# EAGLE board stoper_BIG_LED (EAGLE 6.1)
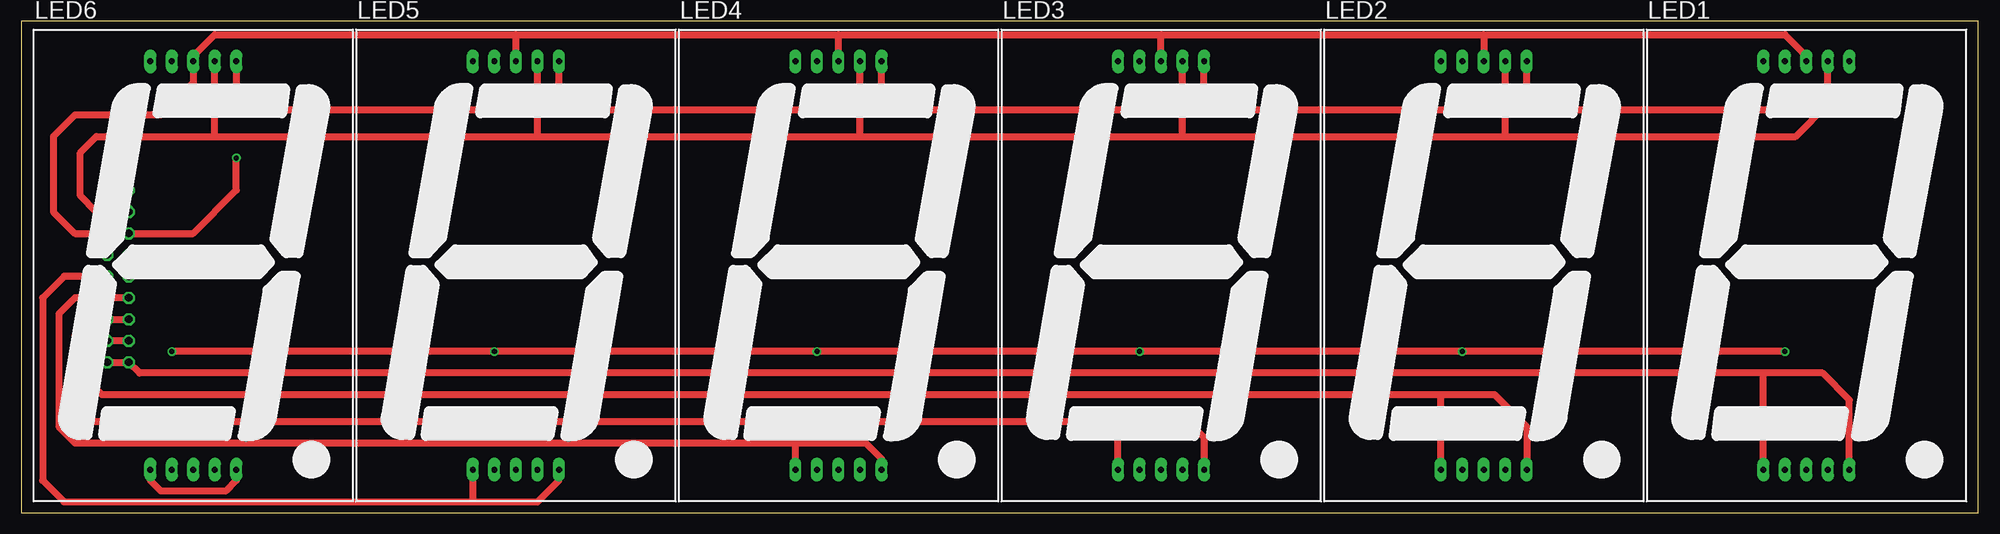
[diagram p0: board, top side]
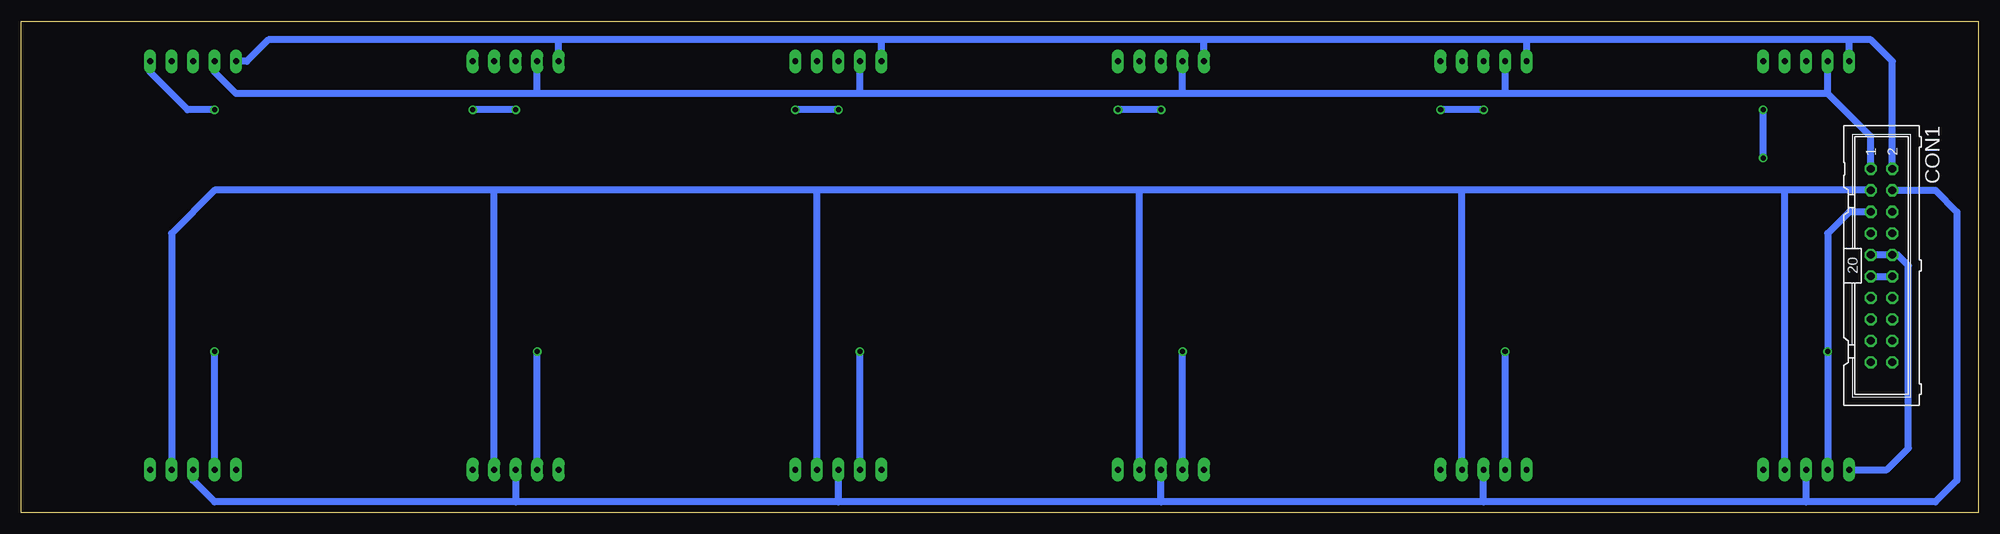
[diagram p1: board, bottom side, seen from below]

Size 231.12 x 58.09 mm. Coordinates in mm from the lower left corner, seen from the top.
Outline: 0,0 231.12,0 231.12,58.09 0,58.09 0,0
Copper layers (1*16): Top 0.035mm / dielectric 1.5mm / Bottom 0.035mm
Design rules: minimum track width 10mil, minimum drill 24mil, track to track 8mil, track to pad 8mil, pad to pad 8mil, via to via 8mil, smd to smd 8mil, copper to edge 40mil, drill to drill 8mil, minimum pad ring 10mil, minimum via ring 8mil, stop-mask expansion 4mil, vias tented up to drill 0mil, thermal gap 10mil

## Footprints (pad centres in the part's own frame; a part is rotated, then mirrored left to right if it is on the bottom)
ML20 = drill 0.914 octagon: 1 -11.43,-1.27; 2 -11.43,1.27; 3 -8.89,-1.27; 4 -8.89,1.27; 5 -6.35,-1.27; 6 -6.35,1.27; 7 -3.81,-1.27; 8 -3.81,1.27; 9 -1.27,-1.27; 10 -1.27,1.27; 11 1.27,-1.27; 12 1.27,1.27; 13 3.81,-1.27; 14 3.81,1.27; 15 6.35,-1.27; 16 6.35,1.27; 17 8.89,-1.27; 18 8.89,1.27; 19 11.43,-1.27; 20 11.43,1.27
SA18-11 = drill 0.7 pad 1.422 long: 1 -5.08,-24.13; 2 -2.54,-24.13; 3 0,-24.13; 4 2.54,-24.13; 5 5.08,-24.13; 6 -5.08,24.13; 7 -2.54,24.13; 8 0,24.13; 9 2.54,24.13; 10 5.08,24.13

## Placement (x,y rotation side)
CON1  [ML20]  11.43,29.21 270 bottom
LED1  7-SEG_SA18-11  [SA18-11]  210.82,29.21 0 top
LED2  7-SEG_SA18-11  [SA18-11]  172.72,29.21 0 top
LED3  7-SEG_SA18-11  [SA18-11]  134.62,29.21 0 top
LED4  7-SEG_SA18-11  [SA18-11]  96.52,29.21 0 top
LED5  7-SEG_SA18-11  [SA18-11]  58.42,29.21 0 top
LED6  7-SEG_SA18-11  [SA18-11]  20.32,29.21 0 top

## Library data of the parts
CON1 = con-harting-ml; OC_FARNELL: unknown; OC_NEWARK: unknown
LED1-LED6 = display-kingbright; OC_FARNELL: unknown; OC_NEWARK: unknown

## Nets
2W1: CON1.19 CON1.20 LED1.1 LED1.5
2W2: CON1.17 CON1.18 LED2.1 LED2.5
2W3: CON1.15 CON1.16 LED3.1 LED3.5
2W4: CON1.13 CON1.14 LED4.1 LED4.5
2W5: CON1.11 CON1.12 LED5.1 LED5.5
2W6: CON1.9 CON1.10 LED6.1 LED6.5
A: CON1.1 LED1.7 LED2.7 LED3.7 LED4.7 LED5.7 LED6.7
B: CON1.2 LED1.6 LED2.6 LED3.6 LED4.6 LED5.6 LED6.6
C: CON1.3 LED1.4 LED2.4 LED3.4 LED4.4 LED5.4 LED6.4
D: CON1.4 LED1.3 LED2.3 LED3.3 LED4.3 LED5.3 LED6.3
DP: CON1.8 LED1.8 LED2.8 LED3.8 LED4.8 LED5.8 LED6.8
E: CON1.5 LED1.2 LED2.2 LED3.2 LED4.2 LED5.2 LED6.2
F: CON1.6 LED1.9 LED2.9 LED3.9 LED4.9 LED5.9 LED6.9
G: CON1.7 LED1.10 LED2.10 LED3.10 LED4.10 LED5.10 LED6.10

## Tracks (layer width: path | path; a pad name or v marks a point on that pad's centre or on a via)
2W1
  Top 0.813: LED1.5 215.9,13.33 212.73,16.51 205.74,16.51 | LED1.1 205.74,16.51 | 205.74,16.51 13.97,16.51 CON1.19 CON1.20
2W2
  Top 0.813: CON1.17 CON1.18 9.53,20.32 8.26,19.05 8.26,15.24 9.53,13.97 167.64,13.97 | 167.64,13.97 173.99,13.97 177.8,10.16 LED2.5 | LED2.1 167.64,13.97
2W3
  Top 0.813: CON1.15 CON1.16 8.26,22.86 6.35,20.95 6.35,12.7 8.26,10.79 129.54,10.79 | 129.54,10.79 137.8,10.79 139.7,8.89 LED3.5 | LED3.1 129.54,10.79
2W4
  Top 0.813: CON1.13 CON1.14 6.35,25.4 4.45,23.5 4.45,10.16 6.35,8.26 91.44,8.26 | 91.44,8.26 99.69,8.26 101.6,6.35 LED4.5 | LED4.1 91.44,8.26
2W5
  Top 0.813: CON1.12 5.08,27.94 2.54,25.4 2.54,3.81 5.08,1.27 53.34,1.27 | 53.34,1.27 60.96,1.27 63.5,3.81 LED5.5 | LED5.1 53.34,1.27
  Bottom 0.813: CON1.11 CON1.12
2W6
  Top 0.813: LED6.5 25.4,3.81 24.13,2.54 16.51,2.54 15.24,3.81 LED6.1
  Bottom 0.813: LED6.1 10.79,5.08 8.26,7.62 8.26,29.21 9.53,30.48 CON1.10 CON1.9
A
  Bottom 0.813: CON1.1 12.7,44.45 17.78,49.53 | 17.78,49.53 LED6.7 | 17.78,49.53 55.88,49.53 | 55.88,49.53 93.98,49.53 | 93.98,49.53 132.08,49.53 | 132.08,49.53 170.18,49.53 | 170.18,49.53 205.74,49.53 208.28,52.07 LED1.7 | 170.18,49.53 LED2.7 | 132.08,49.53 LED3.7 | 93.98,49.53 LED4.7 | 55.88,49.53 LED5.7
B
  Bottom 0.813: CON1.2 10.16,53.34 12.7,55.88 15.24,55.88 | 15.24,55.88 53.34,55.88 | 53.34,55.88 91.44,55.88 | 91.44,55.88 129.54,55.88 | 129.54,55.88 167.64,55.88 | 167.64,55.88 201.93,55.88 204.47,53.34 LED1.6 | LED6.6 15.24,55.88 | LED5.6 53.34,55.88 | LED4.6 91.44,55.88 | LED3.6 129.54,55.88 | LED2.6 167.64,55.88
C
  Bottom 0.813: CON1.3 22.86,38.1 | 22.86,38.1 60.96,38.1 | 60.96,38.1 99.06,38.1 | 99.06,38.1 137.16,38.1 | 137.16,38.1 175.26,38.1 | 175.26,38.1 208.28,38.1 213.36,33.02 LED1.4 | LED2.4 175.26,38.1 | LED3.4 137.16,38.1 | LED4.4 99.06,38.1 | LED5.4 60.96,38.1 | LED6.4 22.86,38.1
D
  Bottom 0.813: CON1.4 5.08,38.1 2.54,35.56 2.54,3.81 5.08,1.27 20.32,1.27 | 20.32,1.27 58.42,1.27 | 58.42,1.27 96.52,1.27 | 96.52,1.27 134.62,1.27 | 134.62,1.27 172.72,1.27 | 172.72,1.27 208.28,1.27 210.82,3.81 LED1.3 | LED2.3 172.72,1.27 | 134.62,1.27 LED3.3 | 96.52,1.27 LED4.3 | 58.42,1.27 LED5.3 | 20.32,1.27 LED6.3
DP
  Top 0.813: CON1.8 6.35,33.02 3.81,35.56 3.81,44.45 6.35,46.99 16.51,46.99 20.32,50.8 LED6.8 20.32,53.98 22.86,56.52 58.42,56.52 | 58.42,56.52 96.52,56.52 | 96.52,56.52 134.62,56.52 | 134.62,56.52 172.72,56.52 | 172.72,56.52 LED2.8 | 172.72,56.52 208.28,56.52 210.82,53.98 LED1.8 | LED3.8 134.62,56.52 | LED4.8 96.52,56.52 | LED5.8 58.42,56.52
E  (via drill 0.6)
  Top 0.813: v17.78,19.05 v55.88,19.05 v93.98,19.05 v132.08,19.05 v170.18,19.05 v208.28,19.05
  Bottom 0.813: CON1.5 15.24,35.56 17.78,33.02 v17.78,19.05 LED6.2 | LED2.2 v170.18,19.05 | LED3.2 v132.08,19.05 | LED4.2 v93.98,19.05 | LED5.2 v55.88,19.05 | LED1.2 v208.28,19.05
F
  Top 0.813: CON1.6 8.89,35.56 6.98,37.47 6.98,42.55 8.89,44.45 22.86,44.45 | 22.86,44.45 LED6.9 | 22.86,44.45 60.96,44.45 | 60.96,44.45 99.06,44.45 | 99.06,44.45 137.16,44.45 | 137.16,44.45 175.26,44.45 | 175.26,44.45 209.55,44.45 213.36,48.26 LED1.9 | 175.26,44.45 LED2.9 | 137.16,44.45 LED3.9 | 60.96,44.45 LED5.9 | 99.06,44.45 LED4.9
G  (via drill 0.6)
  Top 0.813: LED6.10 v25.4,47.62 v58.42,47.62 | LED5.10 v63.5,47.62 v96.52,47.62 | v134.62,47.62 v101.6,47.62 LED4.10 | v172.72,47.62 v139.7,47.62 LED3.10 | v208.28,47.62 v177.8,47.62 LED2.10 | CON1.7 20.32,33.02 25.4,38.1 v25.4,41.91
  Bottom 0.813: v58.42,47.62 v63.5,47.62 | v96.52,47.62 v101.6,47.62 | v134.62,47.62 v139.7,47.62 | v172.72,47.62 v177.8,47.62 | v208.28,47.62 211.46,47.62 215.9,52.07 LED1.10 | v25.4,41.91 v25.4,47.62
